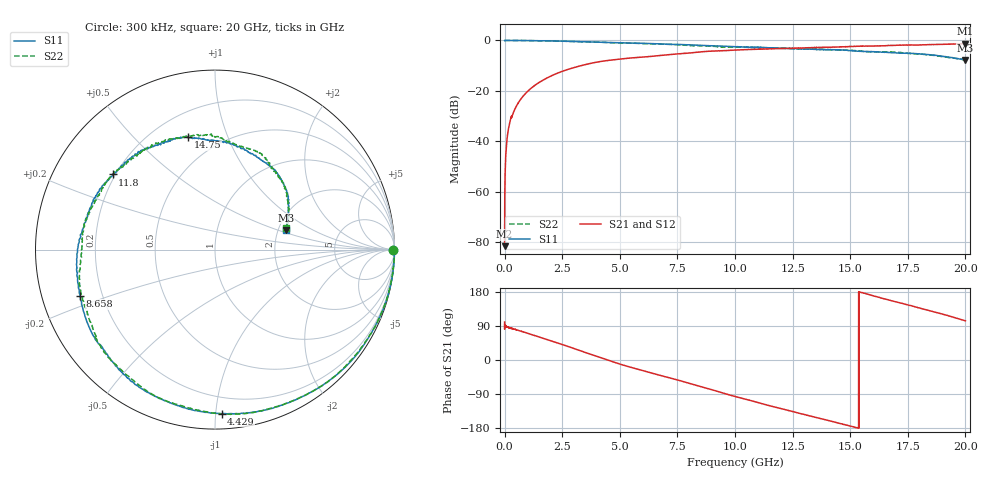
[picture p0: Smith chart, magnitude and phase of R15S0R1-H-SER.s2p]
!{R15S0R1}
!Johanson Technology Inc.
!www.johansontechnology.com
!Test Board Conditions:
!Substrate Type  RO4350B
!Substrate Thickness  20 mil
!Substrate Dk  3.66
!TL Type: GCPW
!TL Trace Width  34 mil
!TL Gap  10 mil
!Electrode orientation  Horizontal
!DUT TOPOLOGY	SERIES
!Mounting Pad LxW  26x52 mil
! Created Sat Feb  6 12:03:19 2021
# hz S ma R 50
! 2 Port Network Data from SP1.SP block
! freq  magS11  angS11  magS21  angS21  magS12  angS12  magS22  angS22
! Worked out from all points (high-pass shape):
!   20001 points, 300 kHz to 20 GHz, reference 50 ohm
!   highest |S21| = -1.28 dB at 19.98 GHz (marker M1); lowest = -81.5 dB at 300 kHz (marker M2)
!   |S21| within 3 dB of the highest: 8.858 GHz to end of sweep
!   lowest |S11| = -7.7 dB at 20 GHz (marker M3), VSWR 2.39, Z = 110 + j29.1 ohm
!   |S11| at or under -10 dB: nowhere
!   |S22| runs from -7.7 to 0.0 dB; largest |S21 - S12| = 0.027
!   S11 on the Smith chart (normalised r, x): 300 kHz: open; 4.429 GHz: 0.09, -1.04; 8.658 GHz: 0.12, -0.16; 11.8 GHz: 0.19, +0.32; 14.75 GHz: 0.34, +0.73; 20 GHz: 2.21, +0.58
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300000  0.9945 0.0  8.399e-05 100.3  6.794e-05 -61.3  0.9937 -0.1
1.033e8  0.999 -2.1  0.011 87.4  0.01097 87.6  0.9999 -2.2
1.483e8  0.9998 -3.1  0.0157 86.4  0.01589 86.5  0.9994 -3.0
2.813e8  0.9989 -6.0  0.02994 83.3  0.02994 83.2  0.9993 -6.0
5.423e8  0.9984 -10.5  0.05293 79.1  0.05305 79.3  0.9981 -10.5
9.523e8  0.9955 -18.3  0.0933 71.3  0.09331 71.3  0.9934 -18.4
1.5163e9  0.9862 -29.7  0.1489 60.2  0.1494 60.1  0.9853 -29.7
2.4713e9  0.9697 -48.3  0.2417 41.3  0.2416 41.3  0.9683 -48.7
3.3343e9  0.9449 -65.8  0.3177 23.5  0.3191 23.5  0.9415 -66.9
4.4293e9  0.9141 -87.7  0.3983 1.0  0.3996 0.9  0.911 -90.1
5.3233e9  0.8913 -104.9  0.443 -16.5  0.442 -16.4  0.8854 -107.6
6.6673e9  0.8567 -128.1  0.4992 -39.2  0.5002 -38.9  0.8471 -129.4
8.6583e9  0.7936 -161.1  0.6009 -72.7  0.6016 -72.5  0.7821 -163.2
1.00003e10  0.7587 175.7  0.6457 -96.2  0.6489 -96.0  0.7443 173.0
1.18033e10  0.707 143.7  0.6888 -125.3  0.691 -125.6  0.71 146.0
1.33343e10  0.671 120.1  0.7223 -148.9  0.7169 -149.1  0.6749 122.4
1.47533e10  0.6443 103.5  0.7481 -170.3  0.7472 -170.5  0.6388 96.1
1.66673e10  0.5777 71.8  0.7954 158.3  0.7904 159.9  0.5967 66.0
1.83293e10  0.527 43.0  0.8243 132.0  0.8303 132.5  0.5231 42.3
1.99813e10  0.4134 15.9  0.8626 103.7  0.8606 104.4  0.4166 17.5
1.99983e10  0.4107 15.5  0.8598 103.5  0.8611 104.1  0.4135 17.1
2e10  0.4111 15.4  0.8594 103.4  0.8624 104.1  0.4129 17.1
